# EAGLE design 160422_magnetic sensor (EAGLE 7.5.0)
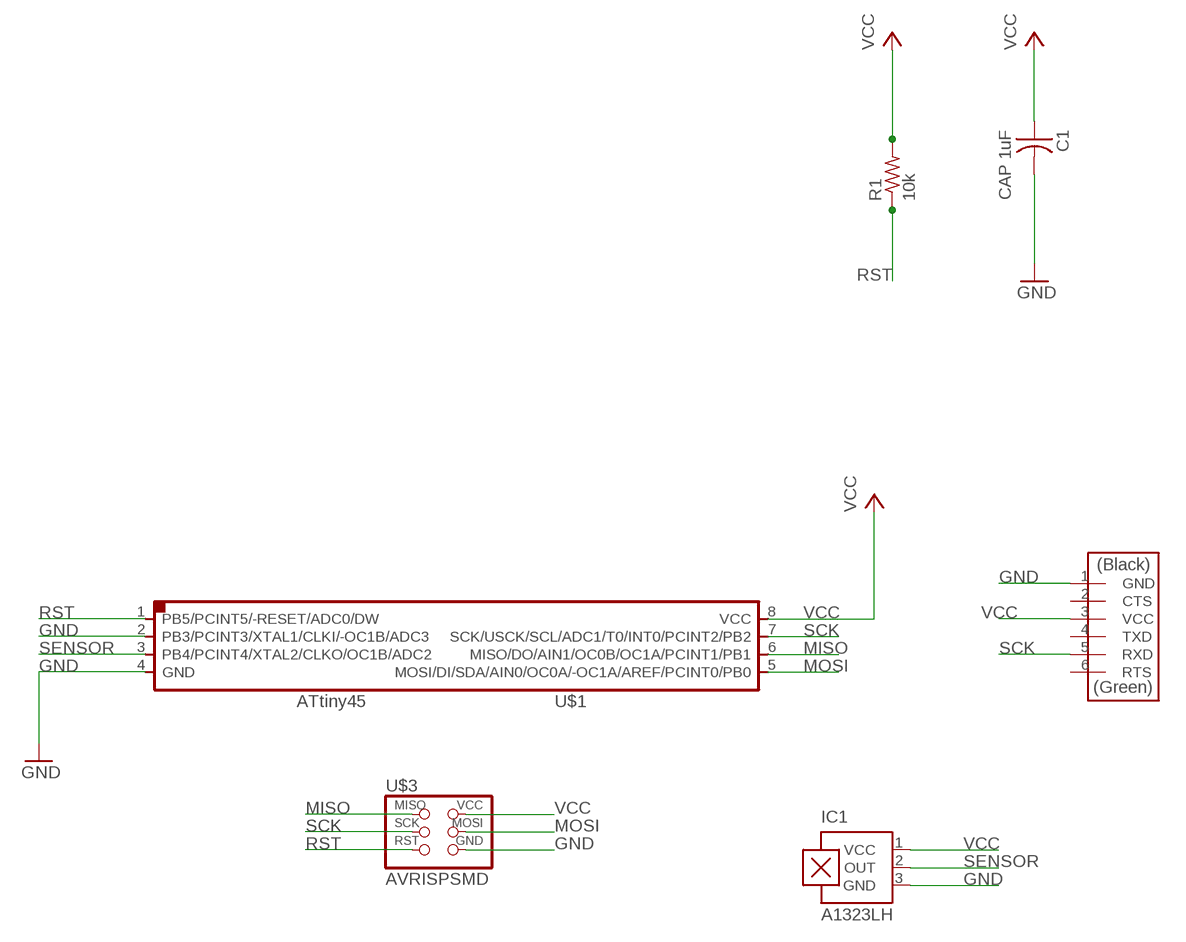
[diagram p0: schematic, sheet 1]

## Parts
C1  CAP 1uF  CAP-US1206FAB  [C1206FAB]
IC1  A1323LH  [SOT23-W]
R1  10k  RES-US1206FAB  [R1206FAB]
U$1  ATTINY45SI  [SOIC8]
U$2  FTDI-SMD-HEADER  [1X06SMD]
U$3  AVRISPSMD  [2X03SMD]

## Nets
GND: C1.2 IC1.3(GND) U$1.2(PB3/PCINT3/XTAL1/CLKI/-OC1B/ADC3) U$1.4(GND) U$2.1(GND) U$3.6(GND)
MISO: U$1.6(MISO/DO/AIN1/OC0B/OC1A/PCINT1/PB1) U$3.1(MISO)
MOSI: U$1.5(MOSI/DI/SDA/AIN0/OC0A/-OC1A/AREF/PCINT0/PB0) U$3.4(MOSI)
RST: R1.1 U$1.1(PB5/PCINT5/-RESET/ADC0/DW) U$3.5(RST)
SCK: U$1.7(SCK/USCK/SCL/ADC1/T0/INT0/PCINT2/PB2) U$2.5(RXD) U$3.3(SCK)
SENSOR: IC1.2(OUT) U$1.3(PB4/PCINT4/XTAL2/CLKO/OC1B/ADC2)
VCC: C1.1 IC1.1(VCC) R1.2 U$1.8(VCC) U$2.3(VCC) U$3.2(VCC)
Unconnected: U$2.2(CTS) U$2.4(TXD) U$2.6(RTS)

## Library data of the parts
C1 = 01-fab:CAP-US
IC1 = allegro:A13*?: Linear Hall Effect Sensor ICs Continuous-Time Ratiometric High-Temperature Operation Programmable Linear with Analog Output A1302 -Replacement- UGN3503 Source: http://www.allegromicro.com/en/Products/Part_Numbers/1301/1301.pdf http://www.allegromicro.com/en/Products/Part_Numbers/1321/1321.pdf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; MF: ALLEGRO MICROSYSTEMS, INC.; MPN: A1323LLHLT-T; OC_FARNELL: 1651968; OC_NEWARK: 65K5152
R1 = 01-fab:RES-US: Resistor (US Symbol)
U$1 = 01-fab:ATTINY45
U$2 = 01-fab:FTDI-SMD-HEADER
U$3 = 01-fab:AVRISP

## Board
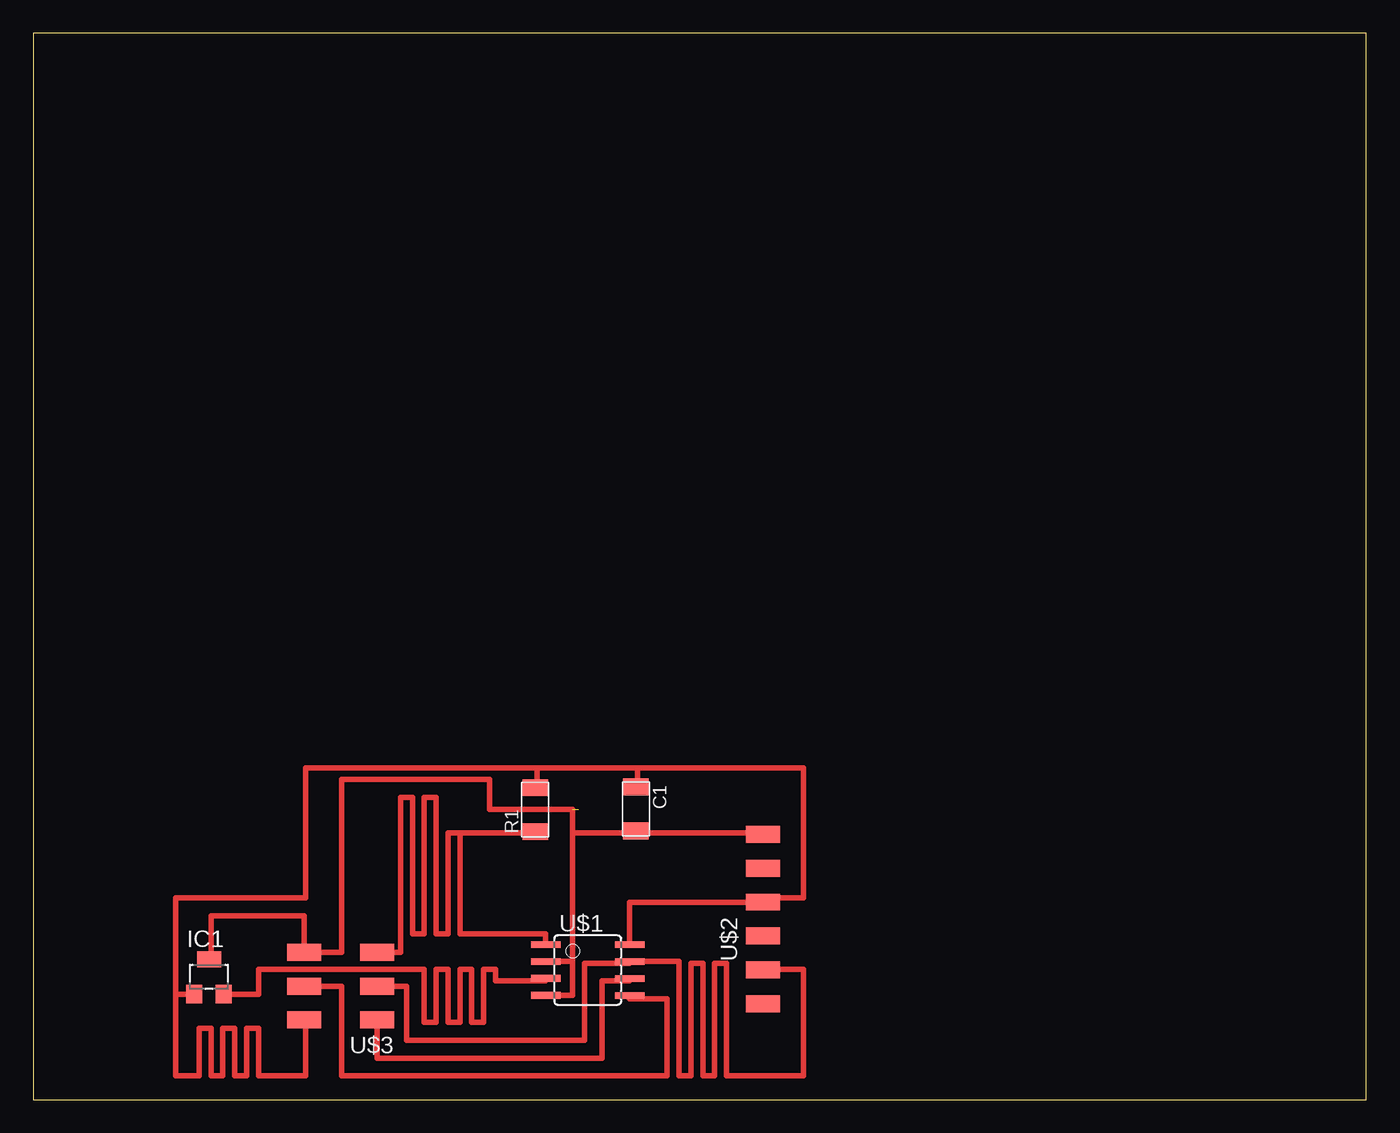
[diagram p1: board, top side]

Size 100 x 80 mm. Coordinates in mm from the lower left corner, seen from the top.
Outline: 0,0 100,0 100,80 0,80 0,0
Copper layers (1*16): Top 0.035mm / dielectric 1.5mm / Bottom 0.035mm
Design rules "default *": minimum track width 10mil, minimum drill 24mil, track to track 16mil, track to pad 16mil, pad to pad 16mil, via to via 16mil, smd to smd 16mil, copper to edge 40mil, drill to drill 8mil, minimum pad ring 10mil, minimum via ring 8mil, stop-mask expansion 4mil, vias tented up to drill 0mil, thermal gap 10mil

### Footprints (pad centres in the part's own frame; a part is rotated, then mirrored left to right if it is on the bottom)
C1206FAB = smd 1.27 x 1.905: 1 -1.651,0; 2 1.651,0
SOT23-W = smd 1.2 x 1.4: 1 -1.1,-1.3; 2 1.1,-1.3 | smd 1.8 x 1.2: 3 0,1.3
R1206FAB = smd 1.27 x 1.905: 1 -1.651,0; 2 1.651,0
SOIC8 = smd 0.5 x 2.2: 1 -1.905,-3.154; 2 -0.645,-3.154; 3 0.625,-3.154; 4 1.895,-3.154; 5 1.905,3.154; 6 0.635,3.154; 7 -0.635,3.154; 8 -1.905,3.154
1X06SMD = smd 2.54 x 1.27: 1 0,6.35; 2 0,3.81; 3 0,1.27; 4 0,-1.27; 5 0,-3.81; 6 0,-6.35
2X03SMD = smd 2.54 x 1.27: 1 -2.54,2.54; 2 2.92,2.54; 3 -2.54,0; 4 2.92,0; 5 -2.54,-2.54; 6 2.92,-2.54

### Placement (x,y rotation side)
C1  45.21,21.81 270 top
IC1  13.18,9.21 0 top
R1  37.66,21.75 90 top
U$1  41.59,9.72 270 top
U$2  54.75,13.54 0 top
U$3  23.24,8.51 180 top

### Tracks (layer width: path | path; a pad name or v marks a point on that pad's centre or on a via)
GND  (1 unrouted)
  Top 0.406: IC1.3 13.34,10.51 13.34,13.78 20.32,13.78 U$3.6 23.11,11.05 23.11,24 34.23,24 34.23,21.78 40.45,21.78 40.45,20 | U$1.4 40.45,7.82 40.45,10.36 | 45.34,20 54.75,20 U$2.1 | C1.2 45.34,20.16 45.34,20 | U$1.2 40.45,10.36 | 40.45,10.36 40.45,20 | 45.34,20 40.45,20
MISO
  Top 0.406: U$3.1 25.78,3.11 42.67,3.11 42.67,8.89 44.75,8.89 U$1.6
MOSI
  Top 0.406: U$1.5 44.75,7.56 47.56,7.56 47.56,1.78 23.11,1.78 23.11,8.51 U$3.4
RST
  Top 0.406: 32,20 31.11,20 31.11,12.45 30.23,12.45 30.23,22.67 29.34,22.67 29.34,12.45 28.45,12.45 28.45,22.67 27.56,22.67 27.56,11.05 U$3.5 | 32,20 32,12.45 38.44,12.45 U$1.1 | 32,20 37.91,20 R1.1
SCK
  Top 0.406: U$3.3 28,8.51 28,4.45 41.34,4.45 41.34,10.22 44.75,10.22 U$1.7 48.45,10.35 48.45,1.78 49.34,1.78 49.34,10.22 50.23,10.22 50.23,1.78 51.12,1.78 51.12,10.22 52.01,10.22 52.01,1.78 57.78,1.78 57.78,9.78 54.75,9.78 U$2.5
SENSOR
  Top 0.406: IC1.2 16.89,7.91 16.89,9.78 29.34,9.78 29.34,5.78 30.23,5.78 30.23,9.78 31.11,9.78 31.11,5.78 32,5.78 32,9.78 32.89,9.78 32.89,5.78 33.78,5.78 33.78,9.78 34.67,9.78 34.67,8.89 38.44,8.89 U$1.3
VCC
  Top 0.406: 20.32,6.22 U$3.2 20.32,5.78 20.45,5.78 20.45,1.78 16.89,1.78 16.89,5.33 16,5.33 16,1.78 15.11,1.78 15.11,5.33 14.22,5.33 14.22,1.78 13.34,1.78 13.34,5.33 12.45,5.33 12.45,1.78 10.67,1.78 10.67,7.91 | 44.45,11.56 44.45,11.62 U$1.8 44.75,14.81 U$2.3 54.75,15.11 57.78,15.11 57.78,24.89 45.34,24.89 | 10.67,7.91 10.67,15.11 20.45,15.11 20.45,24.89 37.78,24.89 | 37.78,24.89 45.34,24.89 | IC1.1 10.67,7.91 | C1.1 45.34,23.46 45.34,24.89 | R1.2 37.78,23.4 37.78,24.89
